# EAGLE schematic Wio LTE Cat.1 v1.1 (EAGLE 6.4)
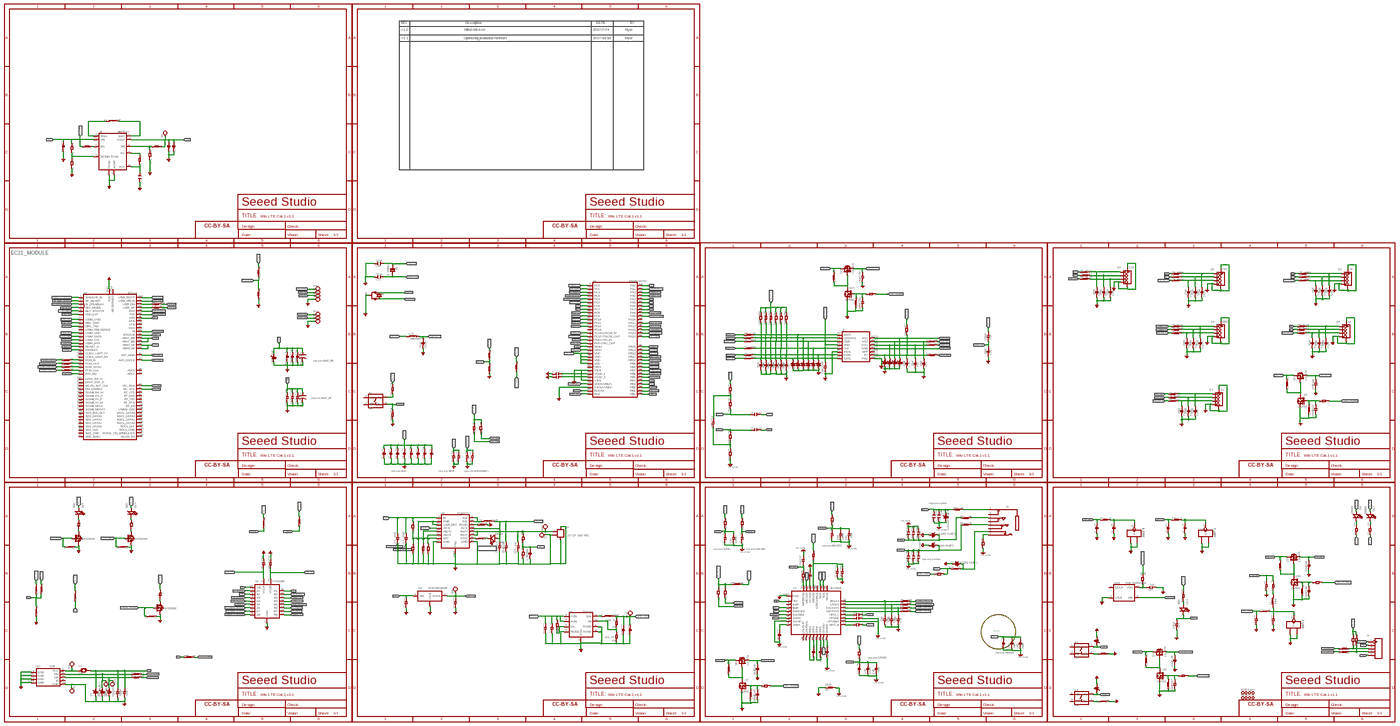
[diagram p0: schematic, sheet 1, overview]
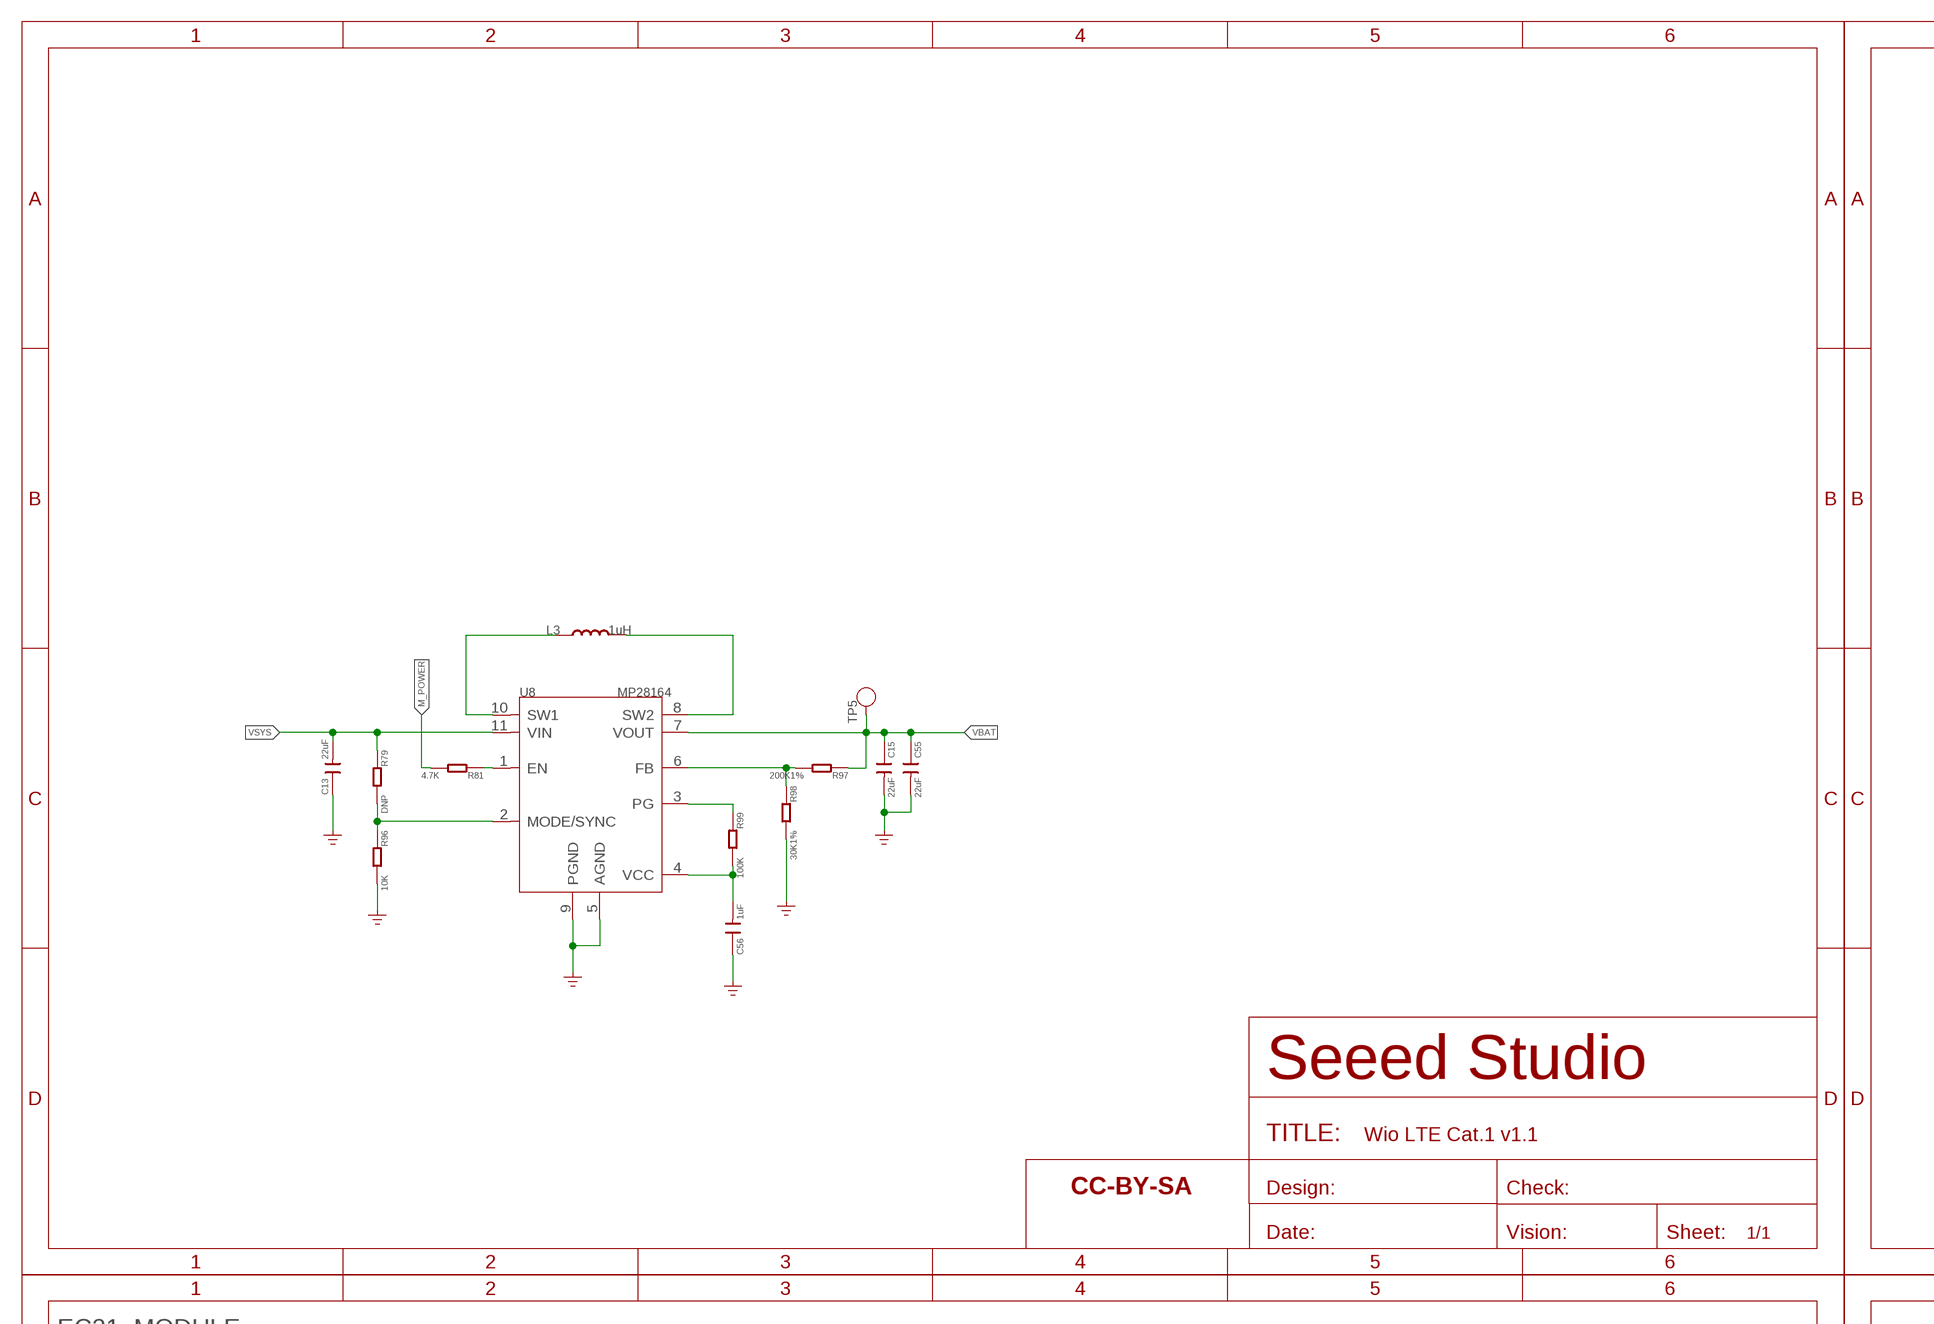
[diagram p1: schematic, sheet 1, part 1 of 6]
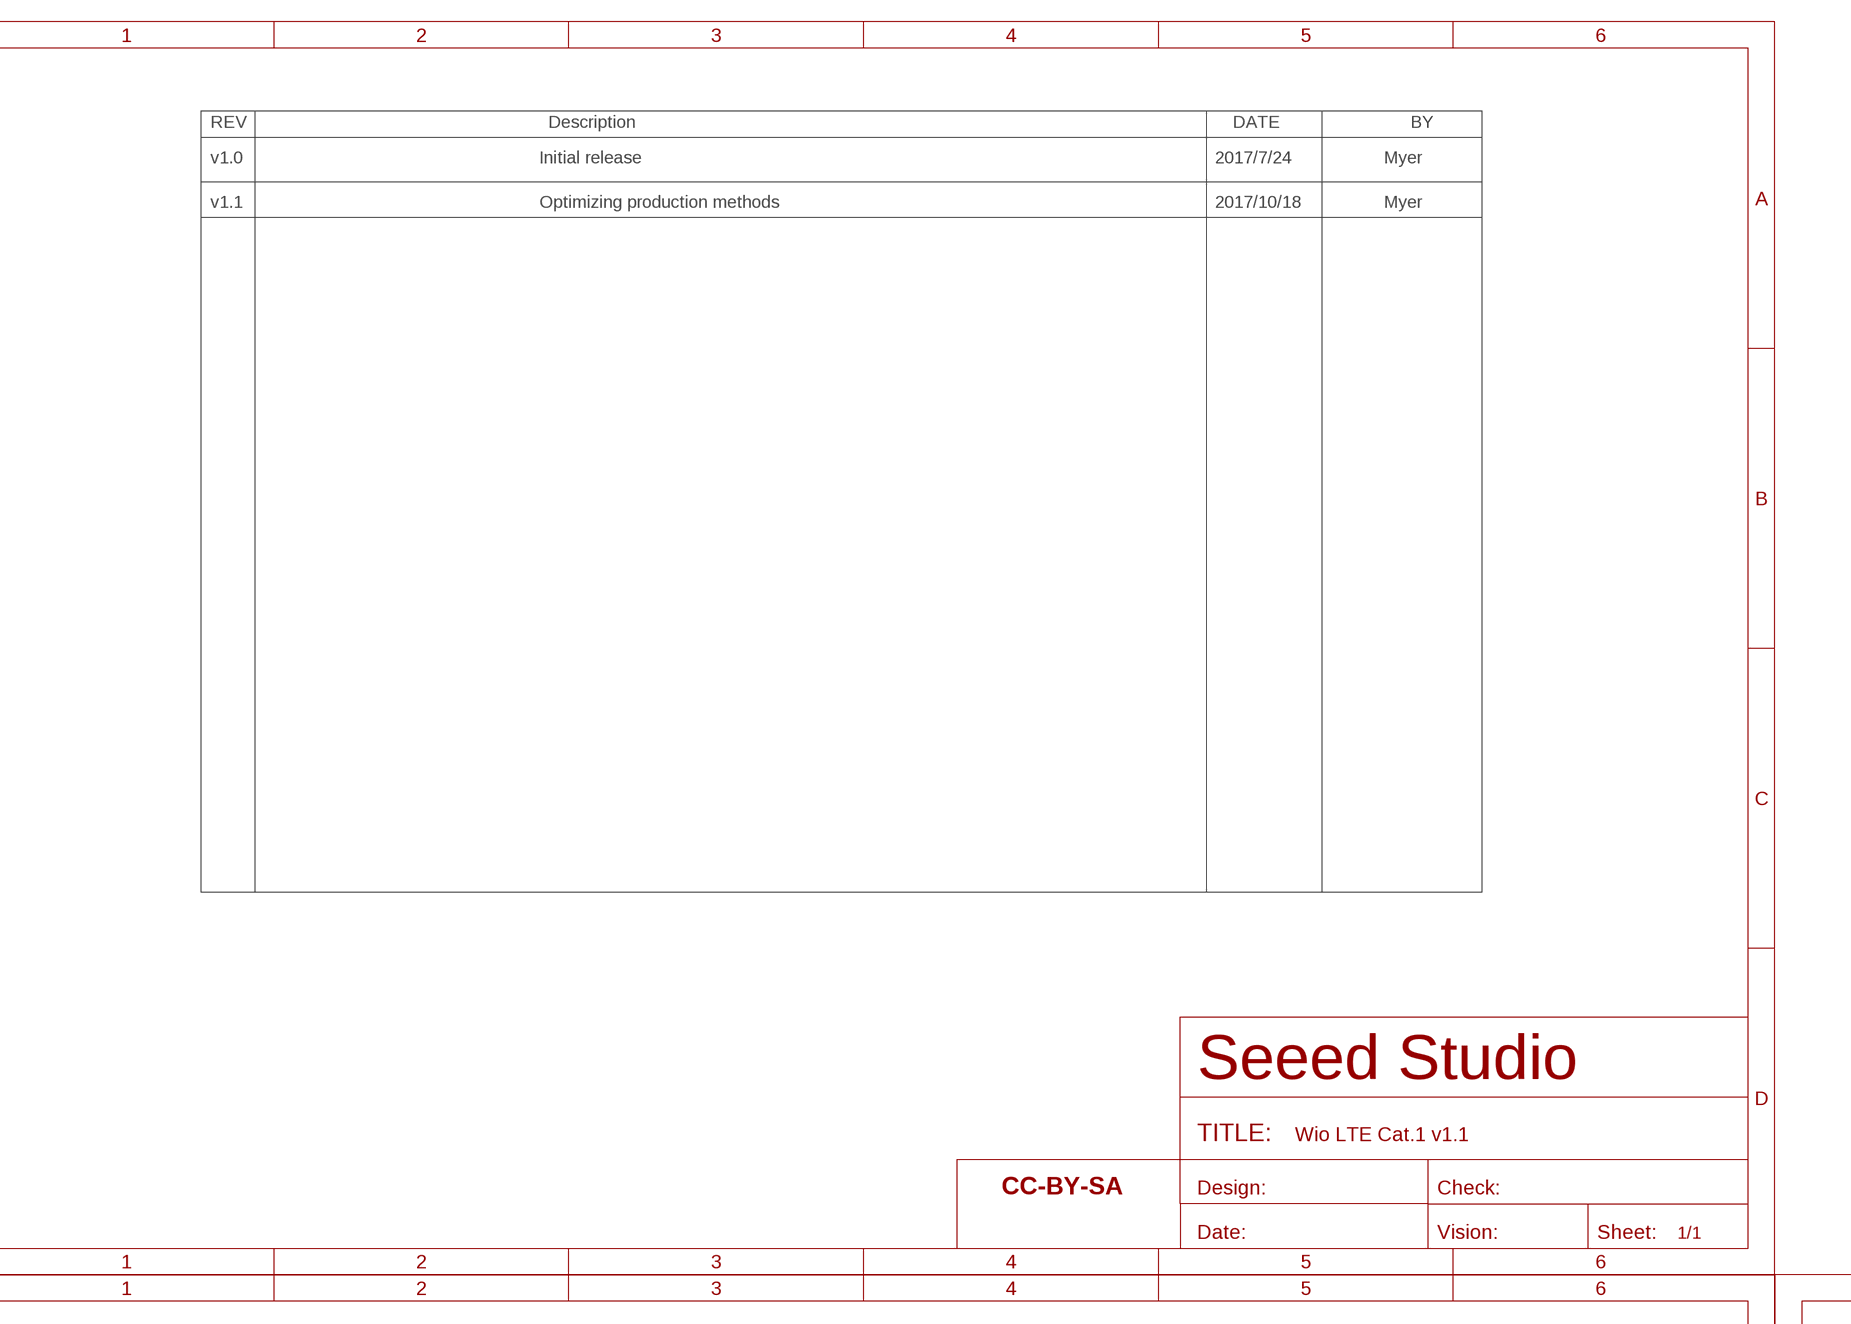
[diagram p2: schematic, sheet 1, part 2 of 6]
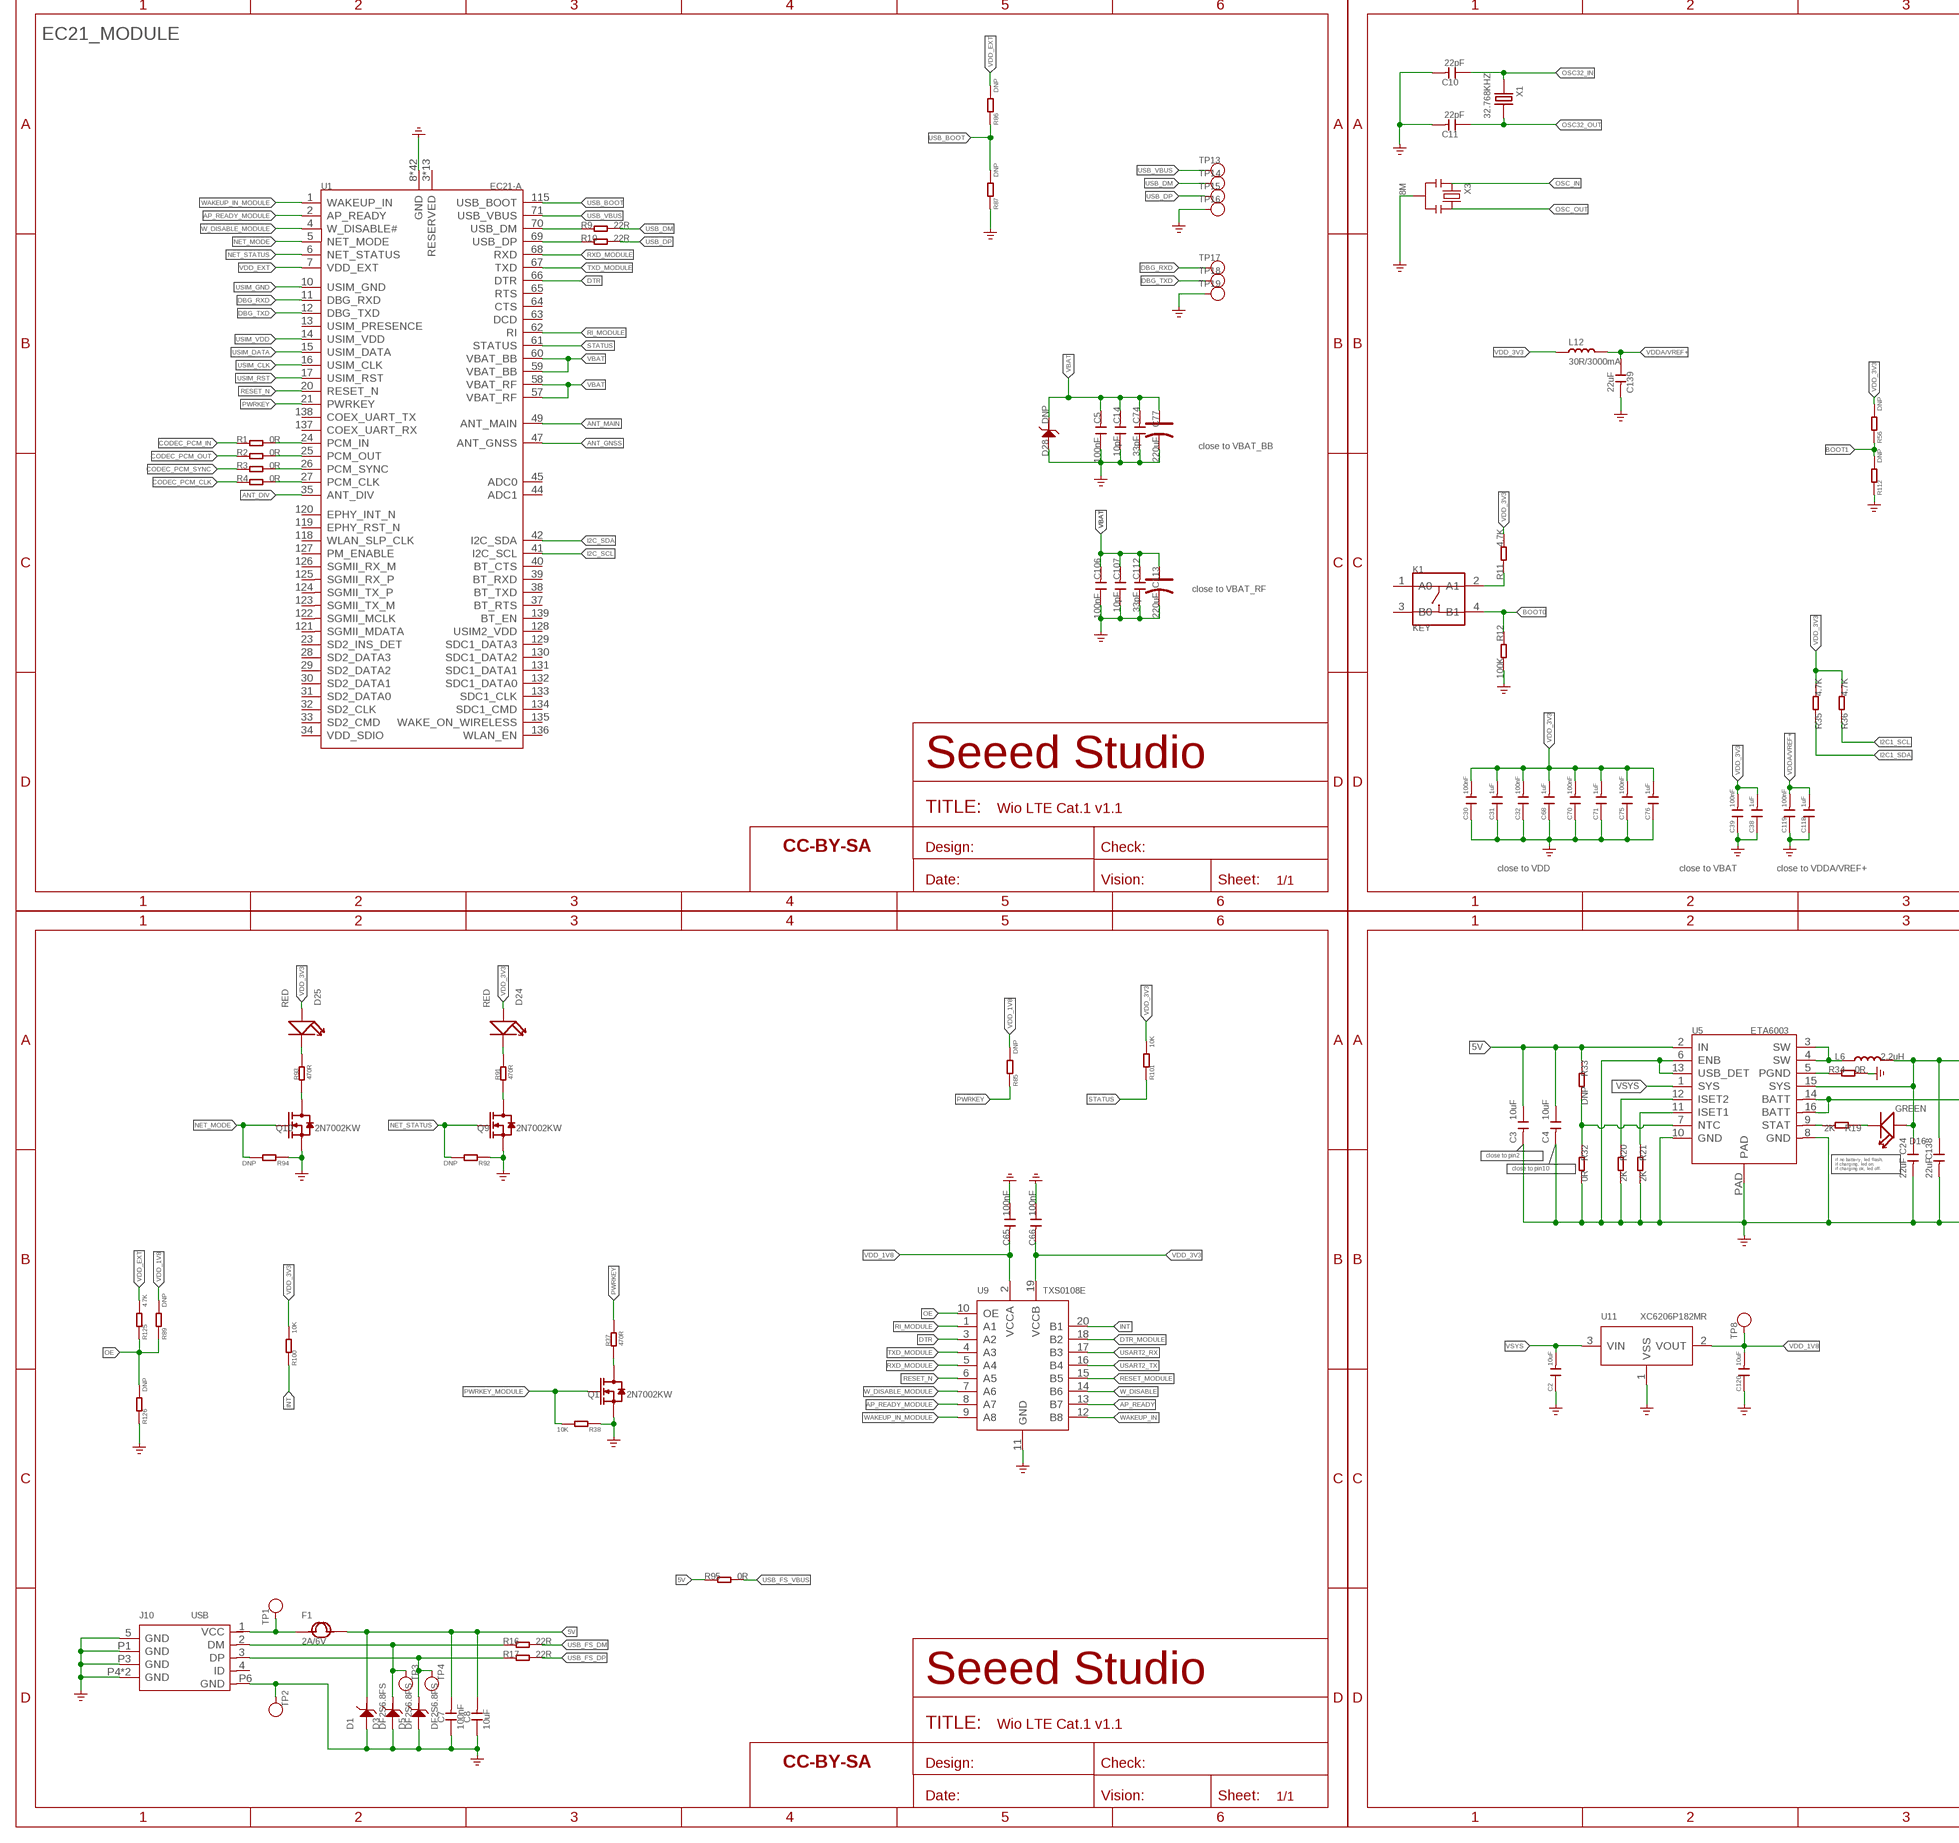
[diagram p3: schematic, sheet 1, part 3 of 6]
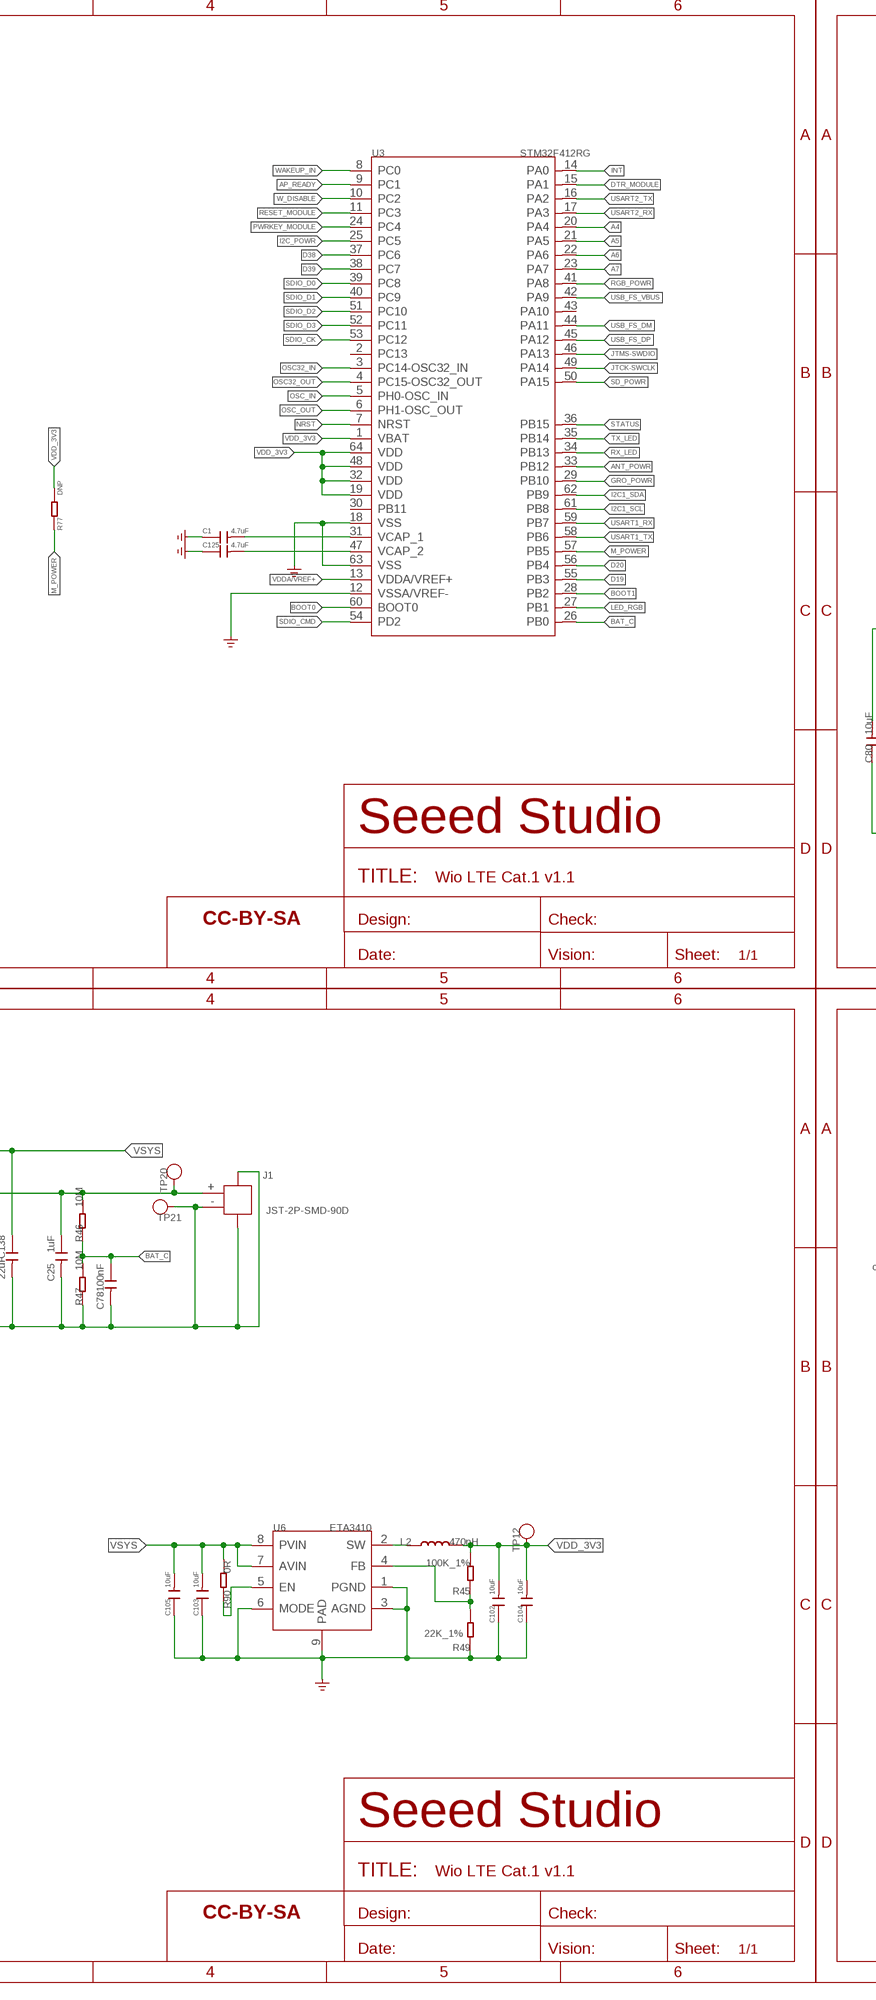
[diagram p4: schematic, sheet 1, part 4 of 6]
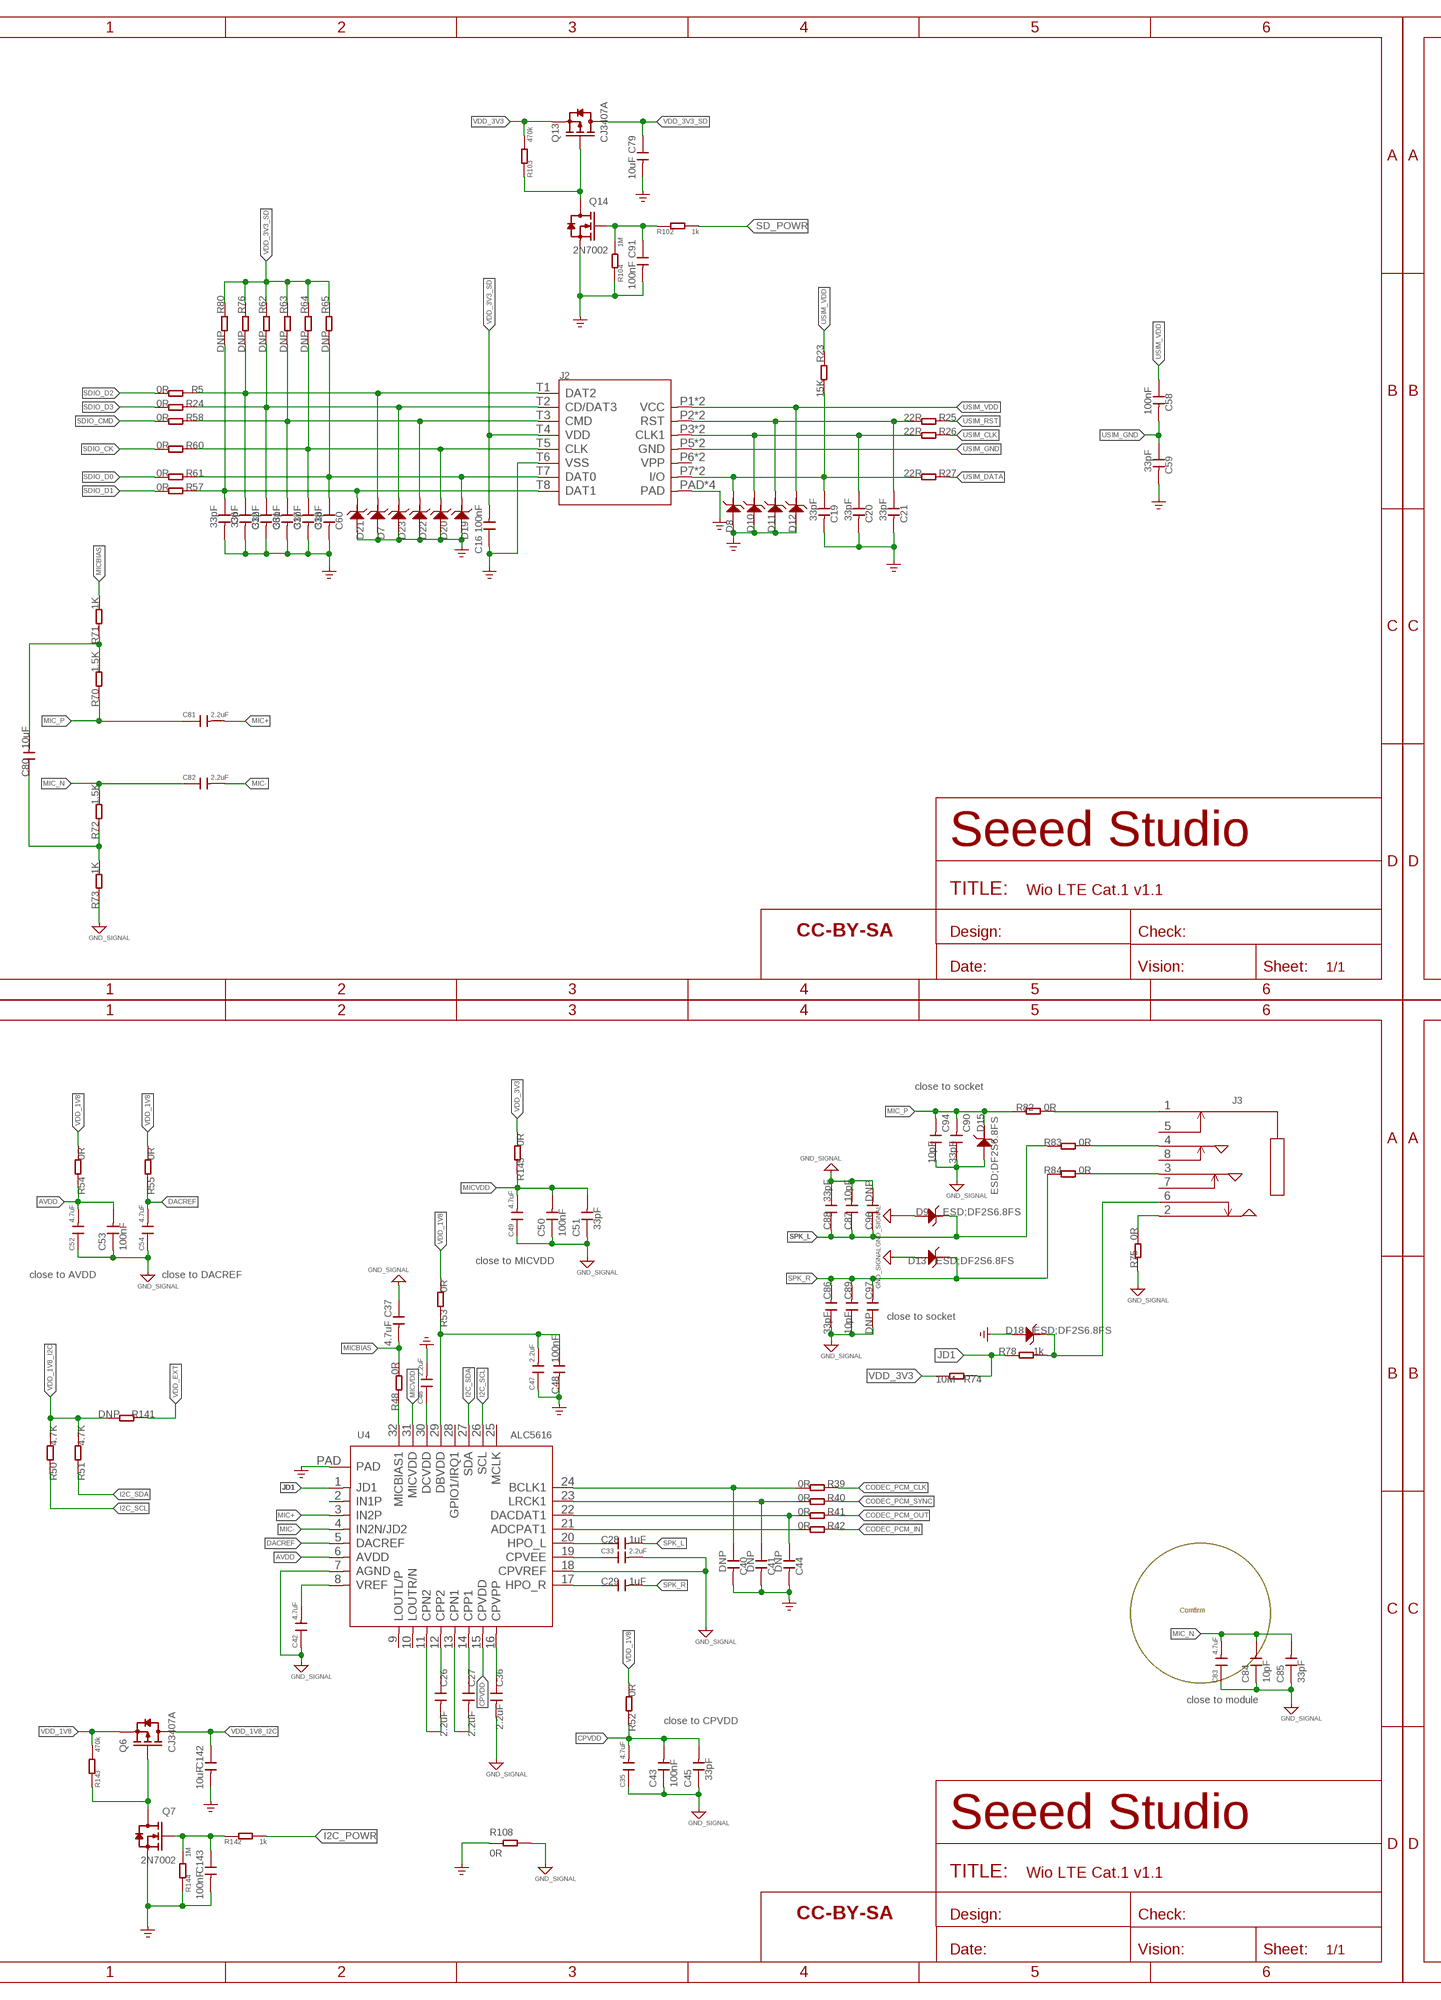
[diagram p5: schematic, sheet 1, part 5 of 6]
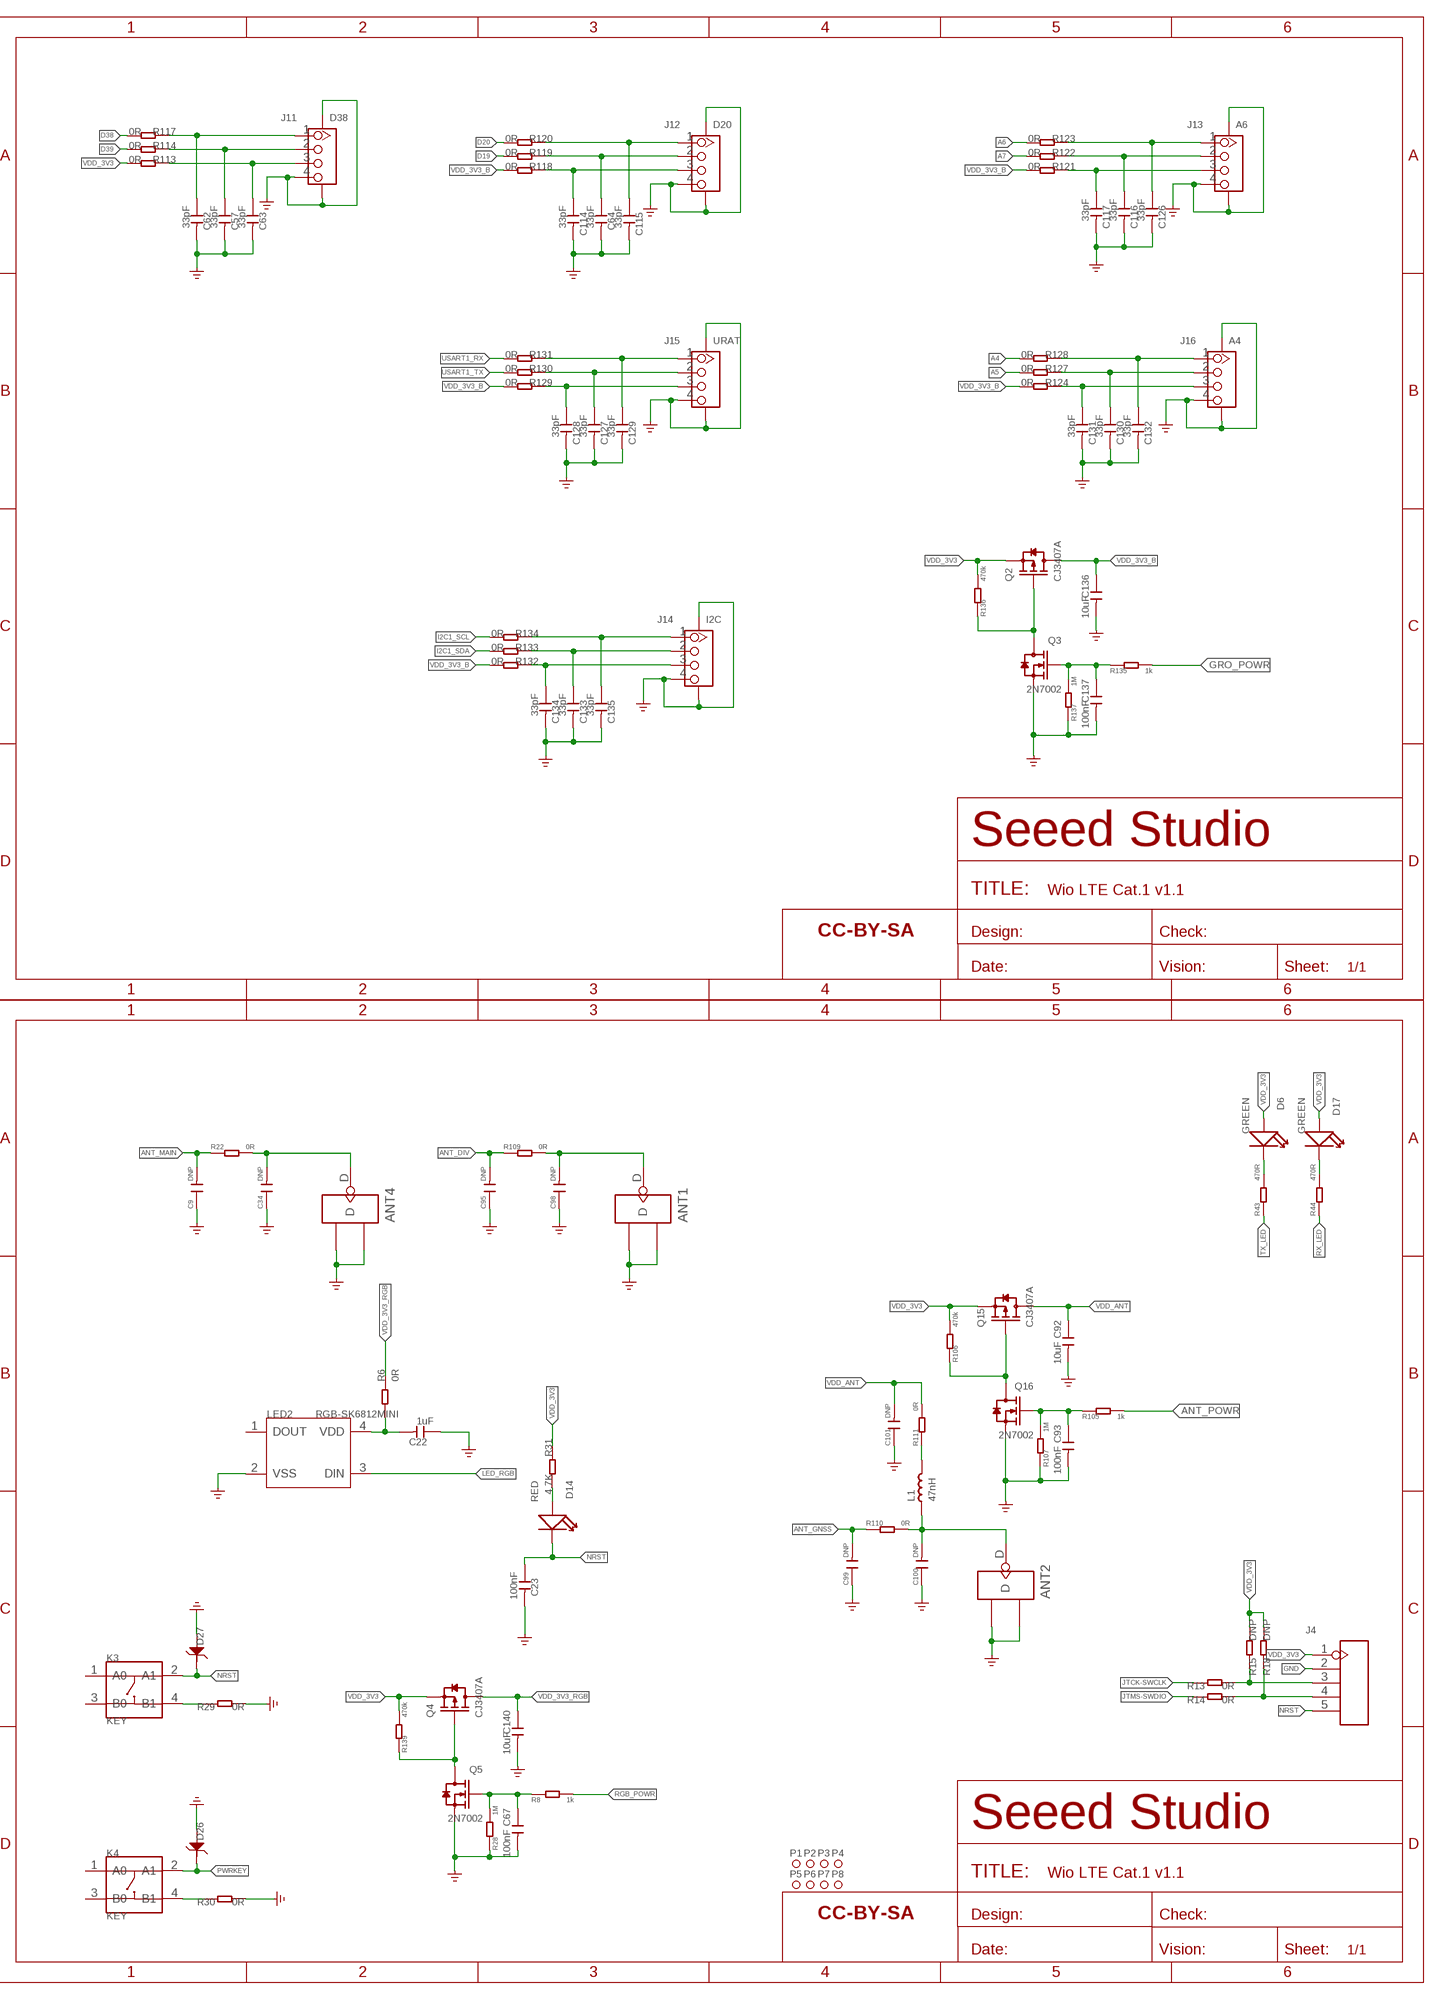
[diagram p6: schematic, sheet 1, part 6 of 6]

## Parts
ANT1  ANTENNA-U-FL  [U-FL3P-SMD-2.6X2.6X1.0MM]
ANT2  ANTENNA-U-FL  [U-FL3P-SMD-2.6X2.6X1.0MM]
ANT4  ANTENNA-U-FL  [U-FL3P-SMD-2.6X2.6X1.0MM]
C1  4.7uF  C-0402  [C0402]
C2  10uF  C-0402  [C0402]
C3  10uF  C-0603  [C0603]
C4  10uF  C-0603  [C0603]
C5  100nF  C-0402  [C0402]
C6  33pF  C-0402  [C0402]
C7  100nF  C-0402  [C0402]
C8  10uF  C-0603  [C0603]
C9  DNP  C-0402  [C0402]
C10  22pF  C-0402  [C0402]
C11  22pF  C-0402  [C0402]
C12  33pF  C-0402  [C0402]
C13  22uF  C-0603  [C0603]
C14  10pF  C-0402  [C0402]
C15  22uF  C-0603  [C0603]
C16  100nF  C-0402  [C0402]
C17  33pF  C-0402  [C0402]
C18  33pF  C-0402  [C0402]
C19  33pF  C-0402  [C0402]
C20  33pF  C-0402  [C0402]
C21  33pF  C-0402  [C0402]
C22  1uF  C-0402  [C0402]
C23  100nF  C-0402  [C0402]
C24  22uF  C-0603  [C0603]
C25  1uF  C-0402  [C0402]
C26  2.2uF  C-0402  [C0402]
C27  2.2uF  C-0402  [C0402]
C28  1uF  C-0603  [C0603]
C29  1uF  C-0603  [C0603]
C30  100nF  C-0402  [C0402]
C31  1uF  C-0402  [C0402]
C32  100nF  C-0402  [C0402]
C33  2.2uF  C-0402  [C0402]
C34  DNP  C-0402  [C0402]
C35  4.7uF  C-0402  [C0402]
C36  2.2uF  C-0402  [C0402]
C37  4.7uF  C-0402  [C0402]
C38  1uF  C-0402  [C0402]
C39  100nF  C-0402  [C0402]
C40  DNP  C-0402  [C0402]
C41  DNP  C-0402  [C0402]
C42  4.7uF  C-0402  [C0402]
C43  100nF  C-0402  [C0402]
C44  DNP  C-0402  [C0402]
C45  33pF  C-0402  [C0402]
C46  2.2uF  C-0402  [C0402]
C47  2.2uF  C-0402  [C0402]
C48  100nF  C-0402  [C0402]
C49  4.7uF  C-0402  [C0402]
C50  100nF  C-0402  [C0402]
C51  33pF  C-0402  [C0402]
C52  4.7uF  C-0402  [C0402]
C53  100nF  C-0402  [C0402]
C54  4.7uF  C-0402  [C0402]
C55  22uF  C-0603  [C0603]
C56  1uF  C-0402  [C0402]
C57  33pF  C-0402  [C0402]
C58  100nF  C-0402  [C0402]
C59  33pF  C-0402  [C0402]
C60  33pF  C-0402  [C0402]
C61  33pF  C-0402  [C0402]
C62  33pF  C-0402  [C0402]
C63  33pF  C-0402  [C0402]
C64  33pF  C-0402  [C0402]
C65  100nF  C-0402  [C0402]
C66  100nF  C-0402  [C0402]
C67  100nF  C-0402  [C0402]
C68  1uF  C-0402  [C0402]
C70  100nF  C-0402  [C0402]
C71  1uF  C-0402  [C0402]
C74  33pF  C-0402  [C0402]
C75  100nF  C-0402  [C0402]
C76  1uF  C-0402  [C0402]
C77  220uF  CAP-POLAR-AVX-B  [AVX-B]
C78  100nF  C-0402  [C0402]
C79  10uF  C-0603  [C0603]
C80  10uF  C-0603  [C0603]
C81  2.2uF  C-0603  [C0603]
C82  2.2uF  C-0603  [C0603]
C83  4.7uF  C-0402  [C0402]
C84  10pF  C-0402  [C0402]
C85  33pF  C-0402  [C0402]
C86  33pF  C-0402  [C0402]
C87  10pF  C-0402  [C0402]
C88  33pF  C-0402  [C0402]
C89  10pF  C-0402  [C0402]
C90  33pF  C-0402  [C0402]
C91  100nF  C-0402  [C0402]
C92  10uF  C-0603  [C0603]
C93  100nF  C-0402  [C0402]
C94  10pF  C-0402  [C0402]
C95  DNP  C-0402  [C0402]
C96  DNP  C-0402  [C0402]
C97  DNP  C-0402  [C0402]
C98  DNP  C-0402  [C0402]
C99  DNP  C-0402  [C0402]
C100  DNP  C-0402  [C0402]
C101  DNP  C-0402  [C0402]
C102  10uF  C-0603  [C0603]
C103  10uF  C-0603  [C0603]
C104  10uF  C-0603  [C0603]
C105  10uF  C-0603  [C0603]
C106  100nF  C-0402  [C0402]
C107  10pF  C-0402  [C0402]
C112  33pF  C-0402  [C0402]
C113  220uF  CAP-POLAR-AVX-B  [AVX-B]
C114  33pF  C-0402  [C0402]
C115  33pF  C-0402  [C0402]
C116  33pF  C-0402  [C0402]
C117  33pF  C-0402  [C0402]
C118  1uF  C-0402  [C0402]
C119  100nF  C-0402  [C0402]
C120  10uF  C-0402  [C0402]
C125  4.7uF  C-0402  [C0402]
C126  33pF  C-0402  [C0402]
C127  33pF  C-0402  [C0402]
C128  33pF  C-0402  [C0402]
C129  33pF  C-0402  [C0402]
C130  33pF  C-0402  [C0402]
C131  33pF  C-0402  [C0402]
C132  33pF  C-0402  [C0402]
C133  33pF  C-0402  [C0402]
C134  33pF  C-0402  [C0402]
C135  33pF  C-0402  [C0402]
C136  10uF  C-0603  [C0603]
C137  100nF  C-0402  [C0402]
C138  22uF  C-0603  [C0603]
C139  22uF  C-0603  [C0603]
C140  10uF  C-0603  [C0603]
C142  10uF  C-0603  [C0603]
C143  100nF  C-0402  [C0402]
D1  DF2S6.8FS  D-ESD-2P'DF2S6.8FS'  [SOD-923]
D3  DF2S6.8FS  D-ESD-2P'DF2S6.8FS'  [SOD-923]
D5  DF2S6.8FS  D-ESD-2P'DF2S6.8FS'  [SOD-923]
D6  GREEN  LED-0402  [LED-0402]
D7  ESD;DF2S6.8FS  D-ESD-2P'DF2S6.8FS'  [SOD-923]
D8  ESD;DF2S6.8FS  D-ESD-2P'DF2S6.8FS'  [SOD-923]
D9  ESD;DF2S6.8FS  D-ESD-2P'DF2S6.8FS'  [SOD-923]
D10  ESD;DF2S6.8FS  D-ESD-2P'DF2S6.8FS'  [SOD-923]
D11  ESD;DF2S6.8FS  D-ESD-2P'DF2S6.8FS'  [SOD-923]
D12  ESD;DF2S6.8FS  D-ESD-2P'DF2S6.8FS'  [SOD-923]
D13  ESD;DF2S6.8FS  D-ESD-2P'DF2S6.8FS'  [SOD-923]
D14  RED  LED-0402  [LED-0402]
D15  ESD;DF2S6.8FS  D-ESD-2P'DF2S6.8FS'  [SOD-923]
D16  GREEN  LED-0402  [LED-0402]
D17  GREEN  LED-0402  [LED-0402]
D18  ESD;DF2S6.8FS  D-ESD-2P'DF2S6.8FS'  [SOD-923]
D19  ESD;DF2S6.8FS  D-ESD-2P'DF2S6.8FS'  [SOD-923]
D20  ESD;DF2S6.8FS  D-ESD-2P'DF2S6.8FS'  [SOD-923]
D21  ESD;DF2S6.8FS  D-ESD-2P'DF2S6.8FS'  [SOD-923]
D22  ESD;DF2S6.8FS  D-ESD-2P'DF2S6.8FS'  [SOD-923]
D23  ESD;DF2S6.8FS  D-ESD-2P'DF2S6.8FS'  [SOD-923]
D24  RED  LED-0402  [LED-0402]
D25  RED  LED-0402  [LED-0402]
D26  ESD;DF2S6.8FS  D-ESD-2P'DF2S6.8FS'  [SOD-923]
D27  ESD;DF2S6.8FS  D-ESD-2P'DF2S6.8FS'  [SOD-923]
D28  DNP  D-ESD-2P'DF2S6.8FS'  [SOD-923]
F1  2A/6V  FUSE'1210'  [F1210]
FR1  SEEEDSTUDIO-OPEN-SCH-FRAME  [SEEEDSTUDIO-PCB-FRAME]
FR2  SEEEDSTUDIO-OPEN-SCH-FRAME  [SEEEDSTUDIO-PCB-FRAME]
FR3  SEEEDSTUDIO-OPEN-SCH-FRAME  [SEEEDSTUDIO-PCB-FRAME]
FR4  SEEEDSTUDIO-OPEN-SCH-FRAME  [SEEEDSTUDIO-PCB-FRAME]
FR5  SEEEDSTUDIO-OPEN-SCH-FRAME  [SEEEDSTUDIO-PCB-FRAME]
FR6  SEEEDSTUDIO-OPEN-SCH-FRAME  [SEEEDSTUDIO-PCB-FRAME]
FR7  SEEEDSTUDIO-OPEN-SCH-FRAME  [SEEEDSTUDIO-PCB-FRAME]
FR8  SEEEDSTUDIO-OPEN-SCH-FRAME  [SEEEDSTUDIO-PCB-FRAME]
FR9  SEEEDSTUDIO-OPEN-SCH-FRAME  [SEEEDSTUDIO-PCB-FRAME]
FR10  SEEEDSTUDIO-OPEN-SCH-FRAME  [SEEEDSTUDIO-PCB-FRAME]
J1  JST-2P-SMD-90D  JST-2P-SMD'1.0'  [HW2-SMD-1.0-90D]
J2  NANO_SIM+TF-24P  [SIM+TF-24P-SMD-1.2-15.05X13.66X2.5MM]
J3  AUDIO-JACK-8P-SMD'PJ-393'  [AUDIO8P-SMD-3.5-14.5X6.1X4.0MM]
J4  HEADER-5P-TEST  [H5-SMD-2.0-TEST]
J10  USB  MICRO-USB5+4P  [MICRO-USB5+5P-SMD-0.65-7.2X5.06MM]
J11  D38  GROVE-CONNECTOR-SMD'90D'  [HW4-SMD-2.0-90D]
J12  D20  GROVE-CONNECTOR-SMD'90D'  [HW4-SMD-2.0-90D]
J13  A6  GROVE-CONNECTOR-SMD'90D'  [HW4-SMD-2.0-90D]
J14  I2C  GROVE-CONNECTOR-SMD'90D'  [HW4-SMD-2.0-90D]
J15  URAT  GROVE-CONNECTOR-SMD'90D'  [HW4-SMD-2.0-90D]
J16  A4  GROVE-CONNECTOR-SMD'90D'  [HW4-SMD-2.0-90D]
K1  KEY  BUTTON-4P-4.5X3.2  [SW4P-SMD-4.5X3.2X2.5MM]
K3  KEY  BUTTON-4P-4.5X3.2  [SW4P-SMD-4.5X3.2X2.5MM]
K4  KEY  BUTTON-4P-4.5X3.2  [SW4P-SMD-4.5X3.2X2.5MM]
L1  47nH  INDUCTOR/FERRITE-BEAD'0402'  [L0402]
L2  470nH  L-MPM201610SR33_T  [L201610]
L3  1uH  L-MPM201610SR33_T  [L201610]
L6  2.2uH  L-MPM201610SR33_T  [L201610]
L12  30R/3000mA  INDUCTOR/FERRITE-BEAD'0603'  [L0603]
LED2  RGB-SK6812MINI  LED-RGB-4P-SK6812-SK6812  [LED4-1.75-3.7X3.5X0.95MM]
P1  MARK-1.0'ANNULAR'  [ROUND-MARK-1.0]
P2  MARK-1.0'ANNULAR'  [ROUND-MARK-1.0]
P3  MARK-1.0'ANNULAR'  [ROUND-MARK-1.0]
P4  MARK-1.0'ANNULAR'  [ROUND-MARK-1.0]
P5  MARK-1.0'ANNULAR'  [ROUND-MARK-1.0]
P6  MARK-1.0'ANNULAR'  [ROUND-MARK-1.0]
P7  MARK-1.0'ANNULAR'  [ROUND-MARK-1.0]
P8  MARK-1.0'ANNULAR'  [ROUND-MARK-1.0]
Q1  2N7002KW  MOSFET-N+'SI1304BDL'  [SOT-323]
Q2  CJ3407A  MOSFET-P'SI2323CDS/SI2305DS<BR>'  [SOT-23]
Q3  2N7002  MOSFET-N+'SOT23'  [SOT-23]
Q4  CJ3407A  MOSFET-P'SI2323CDS/SI2305DS<BR>'  [SOT-23]
Q5  2N7002  MOSFET-N+'SOT23'  [SOT-23]
Q6  CJ3407A  MOSFET-P'SI2323CDS/SI2305DS<BR>'  [SOT-23]
Q7  2N7002  MOSFET-N+'SOT23'  [SOT-23]
Q9  2N7002KW  MOSFET-N+'SI1304BDL'  [SOT-323]
Q10  2N7002KW  MOSFET-N+'SI1304BDL'  [SOT-323]
Q13  CJ3407A  MOSFET-P'SI2323CDS/SI2305DS<BR>'  [SOT-23]
Q14  2N7002  MOSFET-N+'SOT23'  [SOT-23]
Q15  CJ3407A  MOSFET-P'SI2323CDS/SI2305DS<BR>'  [SOT-23]
Q16  2N7002  MOSFET-N+'SOT23'  [SOT-23]
R1  0R  R-0402  [R0402]
R2  0R  R-0402  [R0402]
R3  0R  R-0402  [R0402]
R4  0R  R-0402  [R0402]
R5  0R  R-0402  [R0402]
R6  0R  R-0402  [R0402]
R8  1k  R-0402  [R0402]
R9  22R  R-0402  [R0402]
R10  22R  R-0402  [R0402]
R11  4.7K  R-0402  [R0402]
R12  100K  R-0402  [R0402]
R13  0R  R-0402  [R0402]
R14  0R  R-0402  [R0402]
R15  DNP  R-0402  [R0402]
R16  22R  R-0402  [R0402]
R17  22R  R-0402  [R0402]
R18  DNP  R-0402  [R0402]
R19  2K  R-0402  [R0402]
R20  2K  R-0402  [R0402]
R21  2K  R-0402  [R0402]
R22  0R  R-0402  [R0402]
R23  15K  R-0402  [R0402]
R24  0R  R-0402  [R0402]
R25  22R  R-0402  [R0402]
R26  22R  R-0402  [R0402]
R27  22R  R-0402  [R0402]
R28  1M  R-0402  [R0402]
R29  0R  R-0402  [R0402]
R30  0R  R-0402  [R0402]
R31  4.7K  R-0402  [R0402]
R32  0R  R-0402  [R0402]
R33  DNP  R-0402  [R0402]
R34  0R  R-0402  [R0402]
R35  4.7K  R-0402  [R0402]
R36  4.7K  R-0402  [R0402]
R37  470R  R-0402  [R0402]
R38  10K  R-0402  [R0402]
R39  0R  R-0402  [R0402]
R40  0R  R-0402  [R0402]
R41  0R  R-0402  [R0402]
R42  0R  R-0402  [R0402]
R43  470R  R-0402  [R0402]
R44  470R  R-0402  [R0402]
R45  100K_1%  R-0402  [R0402]
R46  10M  R-0402  [R0402]
R47  10M  R-0402  [R0402]
R48  0R  R-0402  [R0402]
R49  22K_1%  R-0402  [R0402]
R50  4.7K  R-0402  [R0402]
R51  4.7K  R-0402  [R0402]
R52  0R  R-0402  [R0402]
R53  0R  R-0402  [R0402]
R54  0R  R-0402  [R0402]
R55  0R  R-0402  [R0402]
R56  DNP  R-0402  [R0402]
R57  0R  R-0402  [R0402]
R58  0R  R-0402  [R0402]
R60  0R  R-0402  [R0402]
R61  0R  R-0402  [R0402]
R62  DNP  R-0402  [R0402]
R63  DNP  R-0402  [R0402]
R64  DNP  R-0402  [R0402]
R65  DNP  R-0402  [R0402]
R70  1.5K  R-0402  [R0402]
R71  1K  R-0402  [R0402]
R72  1.5K  R-0402  [R0402]
R73  1K  R-0402  [R0402]
R74  10M  R-0402  [R0402]
R75  0R  R-0402  [R0402]
R76  DNP  R-0402  [R0402]
R77  DNP  R-0402  [R0402]
R78  1k  R-0402  [R0402]
R79  DNP  R-0402  [R0402]
R80  DNP  R-0402  [R0402]
R81  4.7K  R-0402  [R0402]
R82  0R  R-0402  [R0402]
R83  0R  R-0603  [R0603]
R84  0R  R-0603  [R0603]
R85  DNP  R-0402  [R0402]
R86  DNP  R-0402  [R0402]
R87  DNP  R-0402  [R0402]
R89  DNP  R-0402  [R0402]
R90  0R  R-0402  [R0402]
R91  470R  R-0402  [R0402]
R92  DNP  R-0402  [R0402]
R93  470R  R-0402  [R0402]
R94  DNP  R-0402  [R0402]
R95  0R  R-0402  [R0402]
R96  10K  R-0402  [R0402]
R97  200K1%  R-0402  [R0402]
R98  30K1%  R-0402  [R0402]
R99  100K  R-0402  [R0402]
R100  10K  R-0402  [R0402]
R101  10K  R-0402  [R0402]
R102  1k  R-0402  [R0402]
R103  470k  R-0402  [R0402]
R104  1M  R-0402  [R0402]
R105  1k  R-0402  [R0402]
R106  470k  R-0402  [R0402]
R107  1M  R-0402  [R0402]
R108  0R  RES-0603  [R0603]
R109  0R  R-0402  [R0402]
R110  0R  R-0402  [R0402]
R111  0R  R-0402  [R0402]
R112  DNP  R-0402  [R0402]
R113  0R  R-0402  [R0402]
R114  0R  R-0402  [R0402]
R117  0R  R-0402  [R0402]
R118  0R  R-0402  [R0402]
R119  0R  R-0402  [R0402]
R120  0R  R-0402  [R0402]
R121  0R  R-0402  [R0402]
R122  0R  R-0402  [R0402]
R123  0R  R-0402  [R0402]
R124  0R  R-0402  [R0402]
R125  4.7K  R-0402  [R0402]
R126  DNP  R-0402  [R0402]
R127  0R  R-0402  [R0402]
R128  0R  R-0402  [R0402]
R129  0R  R-0402  [R0402]
R130  0R  R-0402  [R0402]
R131  0R  R-0402  [R0402]
R132  0R  R-0402  [R0402]
R133  0R  R-0402  [R0402]
R134  0R  R-0402  [R0402]
R135  1k  R-0402  [R0402]
R136  470k  R-0402  [R0402]
R137  1M  R-0402  [R0402]
R139  470k  R-0402  [R0402]
R141  DNP  R-0402  [R0402]
R142  1k  R-0402  [R0402]
R143  470k  R-0402  [R0402]
R144  1M  R-0402  [R0402]
R145  0R  R-0402  [R0402]
TP1  TEST-POINT'4545'  [TP-D45MIL]
TP2  TEST-POINT'4545'  [TP-D45MIL]
TP3  TEST-POINT'4545'  [TP-D45MIL]
TP4  TEST-POINT'4545'  [TP-D45MIL]
TP5  TEST-POINT'4545'  [TP-D45MIL]
TP8  TEST-POINT'4545'  [TP-D45MIL]
TP12  TEST-POINT'4545'  [TP-D45MIL]
TP13  TEST-POINT'4545'  [TP-D45MIL]
TP14  TEST-POINT'4545'  [TP-D45MIL]
TP15  TEST-POINT'4545'  [TP-D45MIL]
TP16  TEST-POINT'4545'  [TP-D45MIL]
TP17  TEST-POINT'4545'  [TP-D45MIL]
TP18  TEST-POINT'4545'  [TP-D45MIL]
TP19  TEST-POINT'4545'  [TP-D45MIL]
TP20  TEST-POINT'4545'  [TP-D45MIL]
TP21  TEST-POINT'4545'  [TP-D45MIL]
U1  EC21-A  MOUDLE-LTE-EC21  [MODULE144P-1.3-32X29X2.4MM]
U3  STM32F412RG  MCU-STM32F412-64P  [LQFP64]
U4  ALC5616  ALC5616  [QFN32G-0.4-4X4MM]
U5  ETA6003  PMIC-ETA6003  [QFN16G-0.5-3X3MM@1]
U6  ETA3410  CONVERTER-ETA3410  [DFN8G-0.5-2X2MM]
U8  MP28164  PMIC-MP28164  [QFN11-0.5-2X3MM]
U9  TXS0108E  LOGIC-TXS0108EPWR  [TSSOP20-0.65-6.5X4.4MM]
U11  XC6206P182MR  PMIC-XC6206PMR  [SOT-23]
X1  32.768KHZ  CRYSTAL-2P'NX2012SA'  [X2-SMD-L2.0X1.2X0.55MM]
X3  8M  CRYSTAL-RESONATOR'SMD'  [RESONATOR3-SMD-3.6X1.3X0.8MM]

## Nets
5V: C3.1 C4.1 C7.2 C8.2 D1.1 F1.2 R33.1 R95.1 U5.2(IN)
A4: R128.2 U3.20(PA4)
A5: R127.2 U3.21(PA5)
A6: R123.2 U3.22(PA6)
A7: R122.2 U3.23(PA7)
AGND: C33.2 C35.1 C36.2 C37.1 C42.1 C43.1 C45.1 C49.1 C50.1 C51.1 C52.1 C53.1 C54.1 C83.1 C84.1 C85.1 C86.1 C87.2 C88.1 C89.1 C90.1 C94.1 C96.2 C97.1 D9.2 D13.2 D15.2 R73.1 R75.1 R108.2 U4.7(AGND) U4.18(CPVREF) ; supply symbol labelled GND_SIGNAL
ANT_DIV: C95.2 R109.1 U1.35(ANT_DIV)
ANT_GNSS: C99.2 R110.1 U1.47(ANT_GNSS)
ANT_MAIN: C9.2 R22.1 U1.49(ANT_MAIN)
ANT_POWR: R105.2 U3.33(PB12)
AP_READY: U3.9(PC1) U9.13(B7)
AP_READY_MODULE: U1.2(AP_READY) U9.8(A7)
AVDD: C52.2 C53.2 R54.1 U4.6(AVDD)
BAT_C: C78.1 R46.1 R47.2 U3.26(PB0)
BOOT0: K1.4(B1) R12.1 U3.60(BOOT0)
BOOT1: R56.1 R112.2 U3.28(PB2)
CD/DATA3: C61.1 D23.1 J2.T2(CD/DAT3) R24.1 R62.2
CODEC_PCM_CLK: R4.1 R39.1
CODEC_PCM_IN: R1.1 R42.1
CODEC_PCM_OUT: R2.1 R41.1
CODEC_PCM_SYNC: R3.1 R40.1
CPVDD: C35.2 C43.2 C45.2 R52.1 U4.15(CPVDD)
D19: R119.2 U3.55(PB3)
D20: R120.2 U3.56(PB4)
D38: R117.2 U3.37(PC6)
D39: R114.2 U3.38(PC7)
DACREF: C54.2 R55.1 U4.5(DACREF)
DBG_RXD: TP17.T U1.11(DBG_RXD)
DBG_TXD: TP18.T U1.12(DBG_TXD)
DTR: U1.66(DTR) U9.3(A2)
DTR_MODULE: U3.15(PA1) U9.18(B2)
GND: ANT1.GND1 ANT1.GND2 ANT2.GND1 ANT2.GND2 ANT4.GND1 ANT4.GND2 C1.1 C2.1 C3.2 C4.2 C5.1 C6.2 C7.1 C8.1 C9.1 C10.2 C11.2 C12.2 C13.1 C14.1 C15.2 C16.1 C17.2 C18.2 C19.2 C20.2 C21.2 C22.1 C23.2 C24.2 C25.2 C30.1 C31.1 C32.1 C34.1 C38.1 C39.1 C40.2 C41.2 C44.2 C46.2 C47.1 C48.2 C55.2 C56.1 C57.2 C59.2 C60.2 C61.2 C62.2 C63.2 C64.2 C65.1 C66.1 C67.2 C68.1 C70.1 C71.1 C74.1 C75.1 C76.1 C77.- C78.2 C79.2 C91.2 C92.2 C93.2 C95.1 C98.1 C99.1 C100.1 C101.1 C102.1 C103.1 C104.1 C105.1 C106.1 C107.1 C112.1 C113.- C114.2 C115.2 C116.2 C117.2 C118.1 C119.1 C120.1 C125.1 C126.2 C127.2 C128.2 C129.2 C130.2 C131.2 C132.2 C133.2 C134.2 C135.2 C136.2 C137.2 C138.2 C139.2 C140.2 C142.2 C143.2 D1.2 D3.2 D5.2 D7.2 D8.2 D10.2 D11.2 D12.2 D18.2 D19.2 D20.2 D21.2 D22.2 D23.2 D26.2 D27.2 D28.2 J1.3 J1.4 J1.- J2.PAD J2.PAD1(PAD) J2.PAD2(PAD) J2.PAD3(PAD) J2.T6(VSS) J4.2 J10.5(GND) J10.P1(GND) J10.P3(GND) J10.P4(GND) J10.P5(GND) J10.P6(GND) J11.4 J11.SS1 J11.SS2 J12.4 J12.SS1 J12.SS2 J13.4 J13.SS1 J13.SS2 J14.4 J14.SS1 J14.SS2 J15.4 J15.SS1 J15.SS2 J16.4 J16.SS1 J16.SS2 LED2.2(VSS) Q1.2(S) Q3.2(S) Q5.2(S) Q7.2(S) Q9.2(S) Q10.2(S) Q14.2(S) Q16.2(S) R12.2 R20.2 R21.2 R28.1 R29.2 R30.2 R32.2 R34.2 R38.1 R47.1 R49.1 R87.1 R92.1 R94.1 R96.2 R98.2 R104.1 R107.1 R108.1 R112.1 R126.1 R137.1 R144.1 TP2.T TP16.T TP19.T TP21.T U1.8(GND) U1.9(GND) U1.19(GND) U1.22(GND) U1.36(GND) U1.46(GND) U1.48(GND) U1.50(GND) U1.51(GND) U1.52(GND) U1.53(GND) U1.54(GND) U1.56(GND) U1.72(GND) U1.85(GND) U1.86(GND) U1.87(GND) U1.88(GND) U1.89(GND) U1.90(GND) U1.91(GND) U1.92(GND) U1.93(GND) U1.94(GND) U1.95(GND) U1.96(GND) U1.97(GND) U1.98(GND) U1.99(GND) U1.100(GND) U1.101(GND) U1.102(GND) U1.103(GND) U1.104(GND) U1.105(GND) U1.106(GND) U1.107(GND) U1.108(GND) U1.109(GND) U1.110(GND) U1.111(GND) U1.112(GND) U3.12(VSSA/VREF-) U3.18(VSS) U3.63(VSS) U4.PAD U5.6(ENB) U5.8(GND) U5.10(GND) U5.13(USB_DET) U5.PAD U6.1(PGND) U6.3(AGND) U6.6(MODE) U6.9(PAD) U8.5(AGND) U8.9(PGND) U9.11(GND) U11.1(VSS) X3.2 ; supply symbol labelled GND_POWER
GRO_POWR: R135.2 U3.29(PB10)
I2C1_SCL: R36.1 R134.2 U3.61(PB8)
I2C1_SDA: R35.1 R133.2 U3.62(PB9)
I2C_POWR: R142.2 U3.25(PC5)
I2C_SCL: R50.1 U1.41(I2C_SCL) U4.26(SCL)
I2C_SDA: R51.1 U1.42(I2C_SDA) U4.27(SDA)
INT: R100.1 U3.14(PA0) U9.20(B1)
JD1: R74.2 R78.1 U4.1(JD1)
JTCK-SWCLK: R13.1 U3.49(PA14)
JTMS-SWDIO: R14.1 U3.46(PA13)
LED_RGB: LED2.3(DIN) U3.27(PB1)
M_POWER: R77.1 R81.2 U3.57(PB5)
MIC+: C81.2 U4.3(IN2P)
MIC-: C82.2 U4.4(IN2N/JD2)
MIC_N: C82.1 C83.2 C84.2 C85.2 R72.2
MIC_P: C81.1 C90.2 C94.2 D15.1 R70.1 R82.1
MICBIAS: C37.2 R48.2 R71.2
MICVDD: C49.2 C50.2 C51.2 R145.1 U4.31(MICVDD)
N$1: R1.2 U1.24(PCM_IN)
N$2: R2.2 U1.25(PCM_OUT)
N$3: R3.2 U1.26(PCM_SYNC)
N$4: R4.2 U1.27(PCM_CLK)
N$5: Q1.3(D) R37.1
N$6: J3.3 R84.2
N$7: R9.1 U1.70(USB_DM)
N$8: R10.1 U1.69(USB_DP)
N$9: D6.- R43.2
N$10: C22.2 LED2.4(VDD) R6.2
N$11: C67.1 Q5.1(G) R8.1 R28.2
N$13: ANT4.D C34.2 R22.2
N$14: D14.+ R31.2
N$15: J3.4 R83.2
N$16: Q4.1(G) Q5.3(D) R139.1
N$17: R90.1 U6.5(EN)
N$18: C1.2 U3.31(VCAP_1)
N$19: C125.2 U3.47(VCAP_2)
N$20: J4.3 R13.2 R15.1
N$21: J4.4 R14.2 R18.1
N$22: D16.- R19.1
N$23: R19.2 U5.9(STAT)
N$24: F1.1 J10.1(VCC) TP1.T
N$25: R32.1 R33.2 U5.7(NTC)
N$26: L6.1 U5.3(SW) U5.4(SW)
N$27: R21.1 U5.11(ISET1)
N$28: C25.1 J1.+ R46.2 TP20.T U5.14(BATT) U5.16(BATT)
N$29: R20.1 U5.12(ISET2)
N$31: K1.2(A1) R11.1
N$33: C12.1 D7.1 J2.T1(DAT2) R5.1 R76.2
N$34: C6.1 D21.1 J2.T8(DAT1) R57.1 R80.2
N$37: L3.1 U8.10(SW1)
N$40: C134.1 J14.3 R132.1
N$41: L3.2 U8.8(SW2)
N$43: C133.1 J14.2 R133.1
N$44: R34.1 U5.5(PGND)
N$45: C135.1 J14.1 R134.1
N$46: R97.2 R98.1 U8.6(FB)
N$47: C63.1 J11.3 R113.1
N$48: L2.1 U6.2(SW)
N$49: R45.1 R49.2 U6.4(FB)
N$50: C28.1 U4.20(HPO_L)
N$51: R81.1 U8.1(EN)
N$52: C57.1 J11.2 R114.1
N$53: D5.1 J10.3(DP) R17.1 TP4.T
N$54: C62.1 J11.1 R117.1
N$55: D3.1 J10.2(DM) R16.1 TP3.T
N$56: D17.- R44.2
N$57: R79.2 R96.1 U8.2(MODE/SYNC)
N$58: R99.1 U8.3(PG)
N$59: C21.1 D11.1 J2.P2(RST) J2.P2B(RST) R25.2
N$60: C20.1 D10.1 J2.P3(CLK1) J2.P3B(CLK1) R26.2
N$61: C56.2 R99.2 U8.4(VCC)
N$62: C19.1 D8.1 J2.P7(I/O) J2.P7B(I/O) R23.2 R27.2
N$63: C114.1 J12.3 R118.1
N$64: C64.1 J12.2 R119.1
N$65: C115.1 J12.1 R120.1
N$66: Q9.3(D) R91.1
N$67: C117.1 J13.3 R121.1
N$68: Q13.1(G) Q14.3(D) R103.1
N$69: C116.1 J13.2 R122.1
N$70: C126.1 J13.1 R123.1
N$71: C128.1 J15.3 R129.1
N$72: C42.2 U4.8(VREF)
N$73: C127.1 J15.2 R130.1
N$74: C129.1 J15.1 R131.1
N$75: C131.1 J16.3 R124.1
N$76: C130.1 J16.2 R127.1
N$77: C132.1 J16.1 R128.1
N$78: C26.2 U4.11(CPN2)
N$79: C26.1 U4.12(CPP2)
N$80: C27.2 U4.13(CPN1)
N$81: C27.1 U4.14(CPP1)
N$82: Q2.1(G) Q3.3(D) R136.1
N$83: C137.1 Q3.1(G) R135.1 R137.2
N$85: C36.1 U4.16(CPVPP)
N$87: Q6.1(G) Q7.3(D) R143.1
N$88: C143.1 Q7.1(G) R142.1 R144.2
N$89: C29.1 U4.17(HPO_R)
N$90: C47.2 C48.1 R53.1 U4.29(DBVDD)
N$93: R42.2 U4.21(ADCPAT1)
N$94: C44.1 R41.2 U4.22(DACDAT1)
N$95: C41.1 R40.2 U4.23(LRCK1)
N$96: C40.1 R39.2 U4.24(BCLK1)
N$97: R48.1 U4.32(MICBIAS1)
N$98: C91.1 Q14.1(G) R102.1 R104.2
N$99: C46.1 U4.30(DCVDD)
N$100: Q15.1(G) Q16.3(D) R106.1
N$105: D24.- R91.2
N$107: C33.1 U4.19(CPVEE)
N$110: Q10.3(D) R93.1
N$111: D25.- R93.2
N$113: C93.1 Q16.1(G) R105.1 R107.2
N$114: ANT1.D C98.2 R109.2
N$115: ANT2.D C100.2 L1.1 R110.2
N$118: L1.2 R111.1
N$120: C80.2 R70.2 R71.1
N$121: C80.1 R72.1 R73.2
N$123: J3.1 R82.2
N$129: K3.4(B1) R29.1
N$130: K4.4(B1) R30.1
N$132: D18.1 J3.6 R78.2
N$134: J3.2 R75.2
NET_MODE: Q10.1(G) R94.2 U1.5(NET_MODE)
NET_STATUS: Q9.1(G) R92.2 U1.6(NET_STATUS)
NRST: C23.1 D14.- D27.1 J4.5 K3.2(A1) U3.7(NRST)
OE: R89.1 R125.1 R126.2 U9.10(OE)
OSC32_IN: C10.1 U3.3(PC14-OSC32_IN) X1.1
OSC32_OUT: C11.1 U3.4(PC15-OSC32_OUT) X1.2
OSC_IN: U3.5(PH0-OSC_IN) X3.1
OSC_OUT: U3.6(PH1-OSC_OUT) X3.3
PWRKEY: D26.1 K4.2(A1) R37.2 R85.1 U1.21(PWRKEY)
PWRKEY_MODULE: Q1.1(G) R38.2 U3.24(PC4)
RESET_MODULE: U3.11(PC3) U9.15(B5)
RESET_N: U1.20(RESET_N) U9.6(A5)
RGB_POWR: R8.2 U3.41(PA8)
RI_MODULE: U1.62(RI) U9.1(A1)
RX_LED: R44.1 U3.34(PB13)
RXD_MODULE: U1.68(RXD) U9.5(A4)
SD_CLK: C18.1 D20.1 J2.T5(CLK) R60.1 R64.2
SD_CMD: C17.1 D22.1 J2.T3(CMD) R58.1 R63.2
SD_DATA0: C60.1 D19.1 J2.T7(DAT0) R61.1 R65.2
SD_POWR: R102.2 U3.50(PA15)
SDIO_CK: R60.2 U3.53(PC12)
SDIO_CMD: R58.2 U3.54(PD2)
SDIO_D0: R61.2 U3.39(PC8)
SDIO_D1: R57.2 U3.40(PC9)
SDIO_D2: R5.2 U3.51(PC10)
SDIO_D3: R24.2 U3.52(PC11)
SPK_L: C28.2 C87.1 C88.2 C96.1 D9.1 R83.1
SPK_R: C29.2 C86.2 C89.2 C97.2 D13.1 R84.1
STATUS: R101.1 U1.61(STATUS) U3.36(PB15)
TX_LED: R43.1 U3.35(PB14)
TXD_MODULE: U1.67(TXD) U9.4(A3)
USART1_RX: R131.2 U3.59(PB7)
USART1_TX: R130.2 U3.58(PB6)
USART2_RX: U3.17(PA3) U9.17(B3)
USART2_TX: U3.16(PA2) U9.16(B4)
USB_BOOT: R86.1 R87.2 U1.115(USB_BOOT)
USB_DM: R9.2 TP14.T
USB_DP: R10.2 TP15.T
USB_FS_DM: R16.2 U3.44(PA11)
USB_FS_DP: R17.2 U3.45(PA12)
USB_FS_VBUS: R95.2 U3.42(PA9)
USB_VBUS: TP13.T U1.71(USB_VBUS)
USIM_CLK: R26.1 U1.16(USIM_CLK)
USIM_DATA: R27.1 U1.15(USIM_DATA)
USIM_GND: C58.2 C59.1 J2.P5(GND) J2.P5B(GND) U1.10(USIM_GND)
USIM_RST: R25.1 U1.17(USIM_RST)
USIM_VDD: C58.1 D12.1 J2.P1(VCC) J2.P1B(VCC) R23.1 U1.14(USIM_VDD)
VBAT: C5.2 C14.2 C15.1 C55.1 C74.2 C77.+ C106.2 C107.2 C112.2 C113.+ D28.1 R97.1 TP5.T U1.57(VBAT_RF) U1.58(VBAT_RF) U1.59(VBAT_BB) U1.60(VBAT_BB) U8.7(VOUT)
VDD_1V8: C65.2 C120.2 Q6.2(S) R52.2 R53.2 R54.2 R55.2 R85.2 R89.2 R143.2 TP8.T U9.2(VCCA) U11.2(VOUT)
VDD_1V8_I2C: C142.1 Q6.3(D) R50.2 R51.2 R141.2
VDD_3V3: C30.2 C31.2 C32.2 C38.2 C39.2 C66.2 C68.2 C70.2 C71.2 C75.2 C76.2 C102.2 C104.2 D6.+ D17.+ D24.+ D25.+ J4.1 L2.2 L12.1 Q2.2(S) Q4.2(S) Q13.2(S) Q15.2(S) R11.2 R15.2 R18.2 R31.1 R35.2 R36.2 R45.2 R56.2 R74.1 R77.2 R100.2 R101.2 R103.2 R106.2 R113.2 R136.2 R139.2 R145.2 TP12.T U3.1(VBAT) U3.19(VDD) U3.32(VDD) U3.48(VDD) U3.64(VDD) U9.19(VCCB)
VDD_3V3_B: C136.1 Q2.3(D) R118.2 R121.2 R124.2 R129.2 R132.2
VDD_3V3_RGB: C140.1 Q4.3(D) R6.1
VDD_3V3_SD: C16.2 C79.1 J2.T4(VDD) Q13.3(D) R62.1 R63.1 R64.1 R65.1 R76.1 R80.1
VDD_ANT: C92.1 C101.2 Q15.3(D) R111.2
VDD_EXT: R86.2 R125.2 R141.1 U1.7(VDD_EXT)
VDDA/VREF+: C118.2 C119.2 C139.1 L12.2 U3.13(VDDA/VREF+)
VSYS: C2.2 C13.2 C24.1 C103.2 C105.2 C138.1 D16.+ L6.2 R79.1 R90.2 U5.1(SYS) U5.15(SYS) U6.7(AVIN) U6.8(PVIN) U8.11(VIN) U11.3(VIN)
W_DISABLE: U3.10(PC2) U9.14(B6)
W_DISABLE_MODULE: U1.4(W_DISABLE#) U9.7(A6)
WAKEUP_IN: U3.8(PC0) U9.12(B8)
WAKEUP_IN_MODULE: U1.1(WAKEUP_IN) U9.9(A8)
Unconnected: J2.P6(VPP) J2.P6B(VPP) J3.5 J3.7 J3.8 J10.4(ID) K1.1(A0) K1.3(B0) K3.1(A0) K3.3(B0) K4.1(A0) K4.3(B0) LED2.1(DOUT) U1.3(RESERVED) U1.13(USIM_PRESENCE) U1.18(RESERVED) U1.23(SD2_INS_DET) U1.28(SD2_DATA3) U1.29(SD2_DATA2) U1.30(SD2_DATA1) U1.31(SD2_DATA0) U1.32(SD2_CLK) U1.33(SD2_CMD) U1.34(VDD_SDIO) U1.37(BT_RTS) U1.38(BT_TXD) U1.39(BT_RXD) U1.40(BT_CTS) U1.43(RESERVED) U1.44(ADC1) U1.45(ADC0) U1.55(RESERVED) U1.63(DCD) U1.64(CTS) U1.65(RTS) U1.113(RESERVED) U1.114(RESERVED) U1.116(RESERVED) U1.117(RESERVED) U1.118(WLAN_SLP_CLK) U1.119(EPHY_RST_N) U1.120(EPHY_INT_N) U1.121(SGMII_MDATA) U1.122(SGMII_MCLK) U1.123(SGMII_TX_M) U1.124(SGMII_TX_P) U1.125(SGMII_RX_P) U1.126(SGMII_RX_M) U1.127(PM_ENABLE) U1.128(USIM2_VDD) U1.129(SDC1_DATA3) U1.130(SDC1_DATA2) U1.131(SDC1_DATA1) U1.132(SDC1_DATA0) U1.133(SDC1_CLK) U1.134(SDC1_CMD) U1.135(WAKE_ON_WIRELESS) U1.136(WLAN_EN) U1.137(COEX_UART_RX) U1.138(COEX_UART_TX) U1.139(BT_EN) U1.140(RESERVED) U1.141(RESERVED) U1.142(RESERVED) U1.143(RESERVED) U1.144(RESERVED) U3.2(PC13) U3.30(PB11) U3.43(PA10) U4.2(IN1P) U4.9(LOUTL/P) U4.10(LOUTR/N) U4.25(MCLK) U4.28(GPIO1/IRQ1)

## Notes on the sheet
- v1.0 | Initial release | 2017/7/24 | Myer
- v1.1 | Optimizing production methods | 2017/10/18 | Myer
- EC21_MODULE
- close to VBAT_BB
- close to VBAT_RF
- close to VDD | close to VBAT | close to VDDA/VREF+
- close to socket
- close to pin2 | close to MICVDD
- close to pin10
- if no battery, led flash.
  if charging, led on.
  if charging ok, led off.
- close to AVDD | close to DACREF
- close to socket
- Comfirm
- close to module
- close to CPVDD

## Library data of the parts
ANT1 ANT2 ANT4 = Connector-new:ANTENNA-U-FL: 320110048
C1-C68 C70 C71 C74-C76 C78-C107 C112 C114-C120 C125-C140 C142 C143 = Discrete-small:C*: Ceramic Capacitors
C77 C113 = Discrete-new:CAP-POLAR: Electrolytic Capacitors,Tantalum Capacitors and Super Capacitors
D1 D3 D5 D7-D13 D15 D18-D23 D26-D28 = Discrete-new:D-ESD-2P: SOD-923:304060009;SOD-123:304060001
D6 D14 D16 D17 D24 D25 = Discrete-new:LED
F1 = Discrete-new:FUSE
FR1-FR10 = moudle-new:SEEEDSTUDIO-OPEN-SCH-FRAME
J1 = Connector-new:JST-2P-SMD: 2P-SMD-1.0-90D:320110054;2P-SMD-2.0-90D:320110026
J2 = Connector-new:NANO_SIM+TF-24P
J3 = Connector-new:AUDIO-JACK-8P-SMD: 320040009
J4 = Connector-new:HEADER-5P
J10 = Connector-new:MICRO-USB5+4P: 5+4P-SMD-0.65-B:320010000;5+2P-SMD-0.65-AB:340032001;5+5P-SMD-0.65-7.2X5.06MM:320010050;
J11-J16 = Connector-new:GROVE-CONNECTOR-SMD: 4P-SMD-2.0:320110030;4P-SMD-2.0-90D:320110032
K1 K3 K4 = Discrete-new:BUTTON-4P: SW4-6.0X6.0X5.0MM:311020024;SW4-8.0X8.0X9.0MM:311020028;SW4-SMD-6.0X6.0X5.0MM:311020004;SW4-SMD-3.35X3.35X1.5MM:311020030;SW4-SMD-5.2X5.2X2.5MM:311020046
L1 L12 = Discrete-new:INDUCTOR/FERRITE-BEAD
L2 L3 L6 = Discrete-new:L
LED2 = Discrete-new:LED-RGB-4P-SK6812
P1-P8 = Discrete-new:MARK-1.0; PARTNO: DNP
Q1 Q3 Q5 Q7 Q9 Q10 Q14 Q16 = Discrete-new:MOSFET-N+: IRLL014: http://www.vishay.com/docs/91319/sihll014.pdf
Q2 Q4 Q6 Q13 Q15 = Discrete-new:MOSFET-P
R1-R6 R8-R58 R60-R65 R70-R87 R89-R107 R109-R114 R117-R137 R139 R141-R145 = Discrete-small:R*
R108 = C-R-package test:RES
TP1-TP5 TP8 TP12-TP21 = Discrete-new:TEST-POINT; PARTNO: DNP
U1 = moudle-new:MOUDLE-LTE-EC21
U3 = IC-new:MCU-STM32F412-64P
U4 = template:ALC5616
U5 = template:PMIC-ETA6003: 2.5A,3MHZ Switching Charger with Dynamic Power Path Management
U6 = IC-new:CONVERTER-ETA3410: 3MHZ 2A High Step-Down Converter in DFN2x2-8L Package
U8 = IC-new:PMIC-MP28164
U9 = IC-new:LOGIC-TXS0108EPWR: 310050026
U11 = IC-new:PMIC-XC6206P: LOW ESR Cap.Compatible Positive Voltage Regulators
X1 = Discrete-new:CRYSTAL-2P
X3 = Discrete-new:CRYSTAL-RESONATOR: Resonator Small SMD resonator. This is the itty bitty 10/20MHz resonators with built in caps. CSTCE10M0G55 and CSTCE20M0V53. Footprint has been reviewed closely but hasn't been tested yet.

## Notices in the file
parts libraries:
moudle-new: This work is licensed under the Creative Commons Attribution 4.0 International License.
To view a copy of this license,visit:
http://creativecommons.org/licenses/by-sa/4.0
moudle-new: CC-BY-SA
